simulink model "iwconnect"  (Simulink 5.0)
settings: Solver=ode45  StartTime=0  StopTime=5  MaxStep=1e-3  RelTol=1e-3
undefined symbols (not defined in the file or in its folder): fro, fso, gamo, vro, wmo
libraries: simulink x5

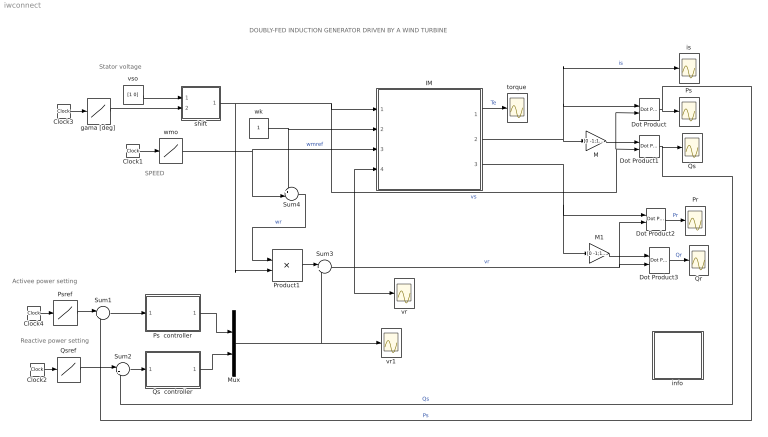
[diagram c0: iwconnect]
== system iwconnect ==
  note: DOUBLY-FED INDUCTION GENERATOR DRIVEN BY A WIND TURBINE
  note: SPEED
  note: Reactive power setting
  note: Activee power setting
  note: Stator voltage
  Clock{1..4} (4 alike) : Clock
  Dot Product{,1..3} (4 alike) : simulink/Math Operations/Dot Product
  IM : Subsystem  mask{Rs=0.01, Lsl=0.1, Rr=0.02, Lm=5, Lrl=0.1, wo=2*pi*60}
      mask prompts: Rs "Stator resistance [pu]"; Lsl "Stator leakage inductance [pu]"; Rr "Rotor resistance [pu]"; Lm "Magnetizing inductance [pu]"; Lrl "Rotor leakage inductance [pu]"; wo "base frequency [rad/s]"
  M : Gain  Gain=[0 -1;1 0]  Multiplication=Matrix(K*u)
  M1 : Gain  Gain=[0 -1;1 0]  Multiplication=Matrix(K*u)
  Mux : Mux  Inputs=2
  Pr : Scope
  Product1 : Product
  Ps : Scope
  Ps  controller : Subsystem  mask{Kp=.07, Ki=10, sat=10}
      mask prompts: Kp "Proportional gain (Kp)"; Ki "Integral gain (Ki)"; sat "Saturation limit [pu]"
      mask help: Proportional-Integral Speed Controller
  Psref : Lookup  InputValues=[0 2 2.01 30 ]  OutputValues=[0 0 -1 -1]
  Qr : Scope
  Qs : Scope
  Qs  controller : Subsystem  mask{Kp=.07, Ki=10, sat=1000}
      mask prompts: Kp "Proportional gain (Kp)"; Ki "Integral gain (Ki)"; sat "Saturation limit [pu]"
      mask help: Proportional-Integral Speed Controller
  Qsref : Lookup  InputValues=[0 3 3.01 10 ]  OutputValues=[0 0 .5 .5]
  Sum1 : Sum  Inputs=|+-
  Sum2 : Sum  Inputs=|++
  Sum3 : Sum  Inputs=|+-
  Sum4 : Sum  Inputs=+-|
  gama [deg] : Lookup  InputValues="[0  1 1.01 20]"  OutputValues=[gamo gamo 20 20]
  info : Subsystem
  is : Scope
  shift : Subsystem
  torque : Scope
  vr : Scope
  vr1 : Scope
  vso : Constant  Value=[1 0]
  wk : Constant
  wmo : Lookup  InputValues=[0 4 4.01 10 ]  OutputValues=[wmo wmo 1.3 1.3]
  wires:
  shift/1(vs) -> IM/1(vs), Dot Product/2, Dot Product1/2, Product1/2  "vs"
  wk/1 -> IM/2(wk), Sum4/1
  Dot Product/1 -> Ps/1, Sum1/2  "Ps"
  M/1 -> Dot Product1/1
  Dot Product1/1 -> Qs/1, Sum2/2  "Qs"
  IM/2(is) -> M/1, Dot Product/1, is/1  "is"
  Dot Product2/1 -> Pr/1  "Pr"
  M1/1 -> Dot Product3/1
  Dot Product3/1 -> Qr/1  "Qr"
  IM/3(ir) -> M1/1, Dot Product2/1
  Clock1/1 -> wmo/1
  wmo/1 -> IM/3(wm), Sum4/2  "wmref"
  IM/1(Te) -> torque/1  "Te"
  Qs  controller/1(Vsqer) -> Mux/2
  Sum2/1 -> Qs  controller/1(Qser)
  Sum1/1 -> Ps  controller/1(Pser)
  Ps  controller/1(Vsder) -> Mux/1
  Sum4/1 -> Product1/1  "wr"
  Product1/1 -> Sum3/1
  Sum3/1 -> IM/4(vr), Dot Product3/2, Dot Product2/2, vr/1  "vr"
  Mux/1 -> vr1/1, Sum3/2
  Clock4/1 -> Psref/1
  Psref/1 -> Sum1/1
  Clock2/1 -> Qsref/1
  Qsref/1 -> Sum2/1
  Clock3/1 -> gama [deg]/1
  vso/1 -> shift/1(vso)
  gama [deg]/1 -> shift/2(gama)

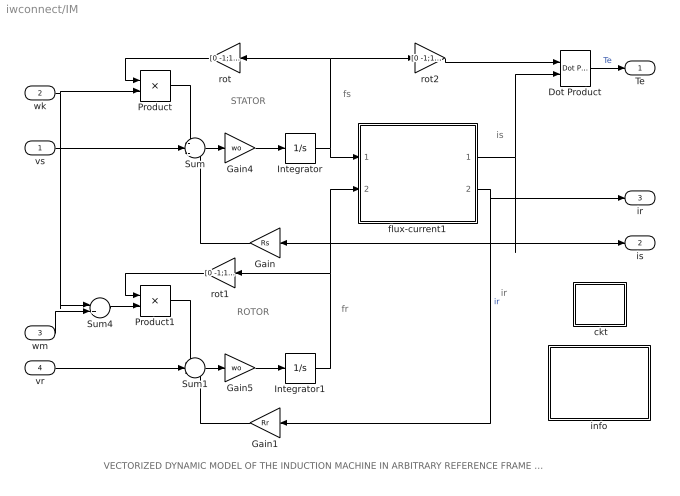
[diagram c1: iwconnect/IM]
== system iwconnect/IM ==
  note: ROTOR
  note: STATOR
  note: fs
  note: fr
  note: is
  note: VECTORIZED DYNAMIC MODEL OF THE INDUCTION MACHINE IN ARBITRARY REFERENCE FRAME (per unit formulation)
  note: ir
  vs : Inport
  wk : Inport  Port=2
  wm : Inport  Port=3
  vr : Inport  Port=4
  " ckt" : Subsystem
  Dot Product : simulink/Math Operations/Dot Product
  Gain : Gain  Orientation=left  Gain=Rs
  Gain1 : Gain  Orientation=left  Gain=Rr
  Gain4 : Gain  Gain=wo
  Gain5 : Gain  Gain=wo
  Integrator : Integrator  InitialCondition=fso
  Integrator1 : Integrator  InitialCondition=fro
  Product : Product
  Product1 : Product
  Sum : Sum  Inputs=-+-
  Sum1 : Sum  Inputs=-+-
  Sum4 : Sum  Inputs=|+-
  flux-current1 : Subsystem
  info : Subsystem
  rot : Gain  Orientation=left  Gain=[0 -1;1 0]  Multiplication=Matrix(K*u)
  rot1 : Gain  Orientation=left  Gain=[0 -1;1 0]  Multiplication=Matrix(K*u)
  rot2 : Gain  Gain=[0 -1;1 0]  Multiplication=Matrix(K*u)
  Te : Outport
  is : Outport  Port=2
  ir : Outport  Port=3
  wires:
  Gain/1 -> Sum/3
  Gain1/1 -> Sum1/3
  flux-current1/2(ir) -> Gain1/1, ir/1  "ir"
  Integrator/1 -> flux-current1/1(fs), rot/1, rot2/1
  Integrator1/1 -> flux-current1/2(fr), rot1/1
  Product1/1 -> Sum1/1
  rot1/1 -> Product1/1
  Product/1 -> Sum/1
  rot/1 -> Product/1
  rot2/1 -> Dot Product/1
  Sum4/1 -> Product1/2
  Sum/1 -> Gain4/1
  Gain4/1 -> Integrator/1
  Sum1/1 -> Gain5/1
  Gain5/1 -> Integrator1/1
  flux-current1/1(is) -> Gain/1, is/1, Dot Product/2
  Dot Product/1 -> Te/1  "Te"
  vs/1 -> Sum/2
  wk/1 -> Product/2, Sum4/1
  wm/1 -> Sum4/2
  vr/1 -> Sum1/2

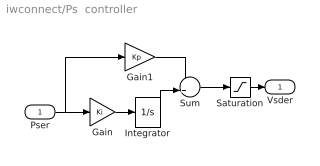
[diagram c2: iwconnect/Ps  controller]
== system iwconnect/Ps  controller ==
  Pser : Inport
  Gain : Gain  Gain=Ki
  Gain1 : Gain  Gain=Kp
  Integrator : Integrator  InitialCondition=vro(1)  LimitOutput=on  UpperSaturationLimit=sat  LowerSaturationLimit=-sat
  Saturation : Saturate  UpperLimit=sat  LowerLimit=-sat
  Sum : Sum
  Vsder : Outport  InitialOutput=0
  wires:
  Integrator/1 -> Sum/2
  Gain1/1 -> Sum/1
  Gain/1 -> Integrator/1
  Pser/1 -> Gain/1, Gain1/1
  Sum/1 -> Saturation/1
  Saturation/1 -> Vsder/1

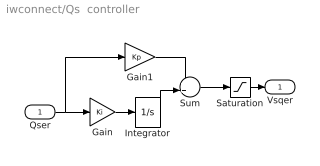
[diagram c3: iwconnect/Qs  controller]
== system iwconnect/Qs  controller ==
  Qser : Inport
  Gain : Gain  Gain=Ki
  Gain1 : Gain  Gain=Kp
  Integrator : Integrator  InitialCondition=vro(2)  LimitOutput=on  UpperSaturationLimit=sat  LowerSaturationLimit=-sat
  Saturation : Saturate  UpperLimit=sat  LowerLimit=-sat
  Sum : Sum
  Vsqer : Outport  InitialOutput=0
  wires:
  Saturation/1 -> Vsqer/1
  Sum/1 -> Saturation/1
  Qser/1 -> Gain1/1, Gain/1
  Gain/1 -> Integrator/1
  Gain1/1 -> Sum/1
  Integrator/1 -> Sum/2

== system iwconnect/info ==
  note: The induction machine is modeled in vectorized form in the synchronous frame . The d-axis is aligned with the stator space voltage vector. The injected rotor voltages (at slip frequency) are derived from PI controllers that regulate the active and reactive powers delivered by the generator. The speed is adjusted by the turbine pitch control to maximize the power generated at a given wind speed. The whole system is described by parameters expressed in per unit. The machine representations are based on the motor convention; consequently in the generator mode of operation, such quantities as Ps, Qs, Tw, Te are negative (with wm>0) while Pr is positive for subsynchronous operation and negative for oversynchronous mode. Before running this model, must be run in order to establish the initial conditions when the generator stator is disconnected from the grid.
  note: Doubly-Fed Induction Generator driven by a Wind Turbine

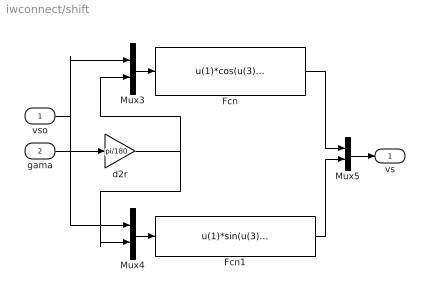
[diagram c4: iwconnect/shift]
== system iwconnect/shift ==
  vso : Inport
  gama : Inport  Port=2
  Fcn : Fcn  Expr=u(1)*cos(u(3))-u(2)*sin(u(3))
  Fcn1 : Fcn  Expr=u(1)*sin(u(3))+u(2)*cos(u(3))
  Mux3 : Mux  Inputs=2
  Mux4 : Mux  Inputs=2
  Mux5 : Mux  Inputs=2
  d2r : Gain  Gain=pi/180  Multiplication=Matrix(K*u)
  vs : Outport
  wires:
  Mux5/1 -> vs/1
  Fcn/1 -> Mux5/1
  Fcn1/1 -> Mux5/2
  gama/1 -> d2r/1
  vso/1 -> Mux4/1, Mux3/1
  Mux4/1 -> Fcn1/1
  Mux3/1 -> Fcn/1
  d2r/1 -> Mux4/2, Mux3/2

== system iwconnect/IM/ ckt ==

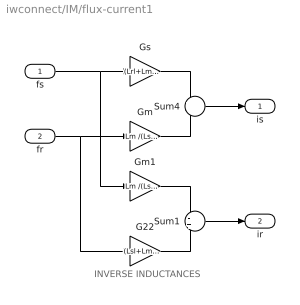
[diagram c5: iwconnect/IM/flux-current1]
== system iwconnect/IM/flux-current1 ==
  note: INVERSE INDUCTANCES
  fs : Inport
  fr : Inport  Port=2
  G22 : Gain  Gain=(Lsl+Lm )/(Lsl*Lrl+Lsl*Lm+Lrl*Lm)
  Gm : Gain  Gain=Lm /(Lsl*Lrl+Lsl*Lm+Lrl*Lm)
  Gm1 : Gain  Gain=Lm /(Lsl*Lrl+Lsl*Lm+Lrl*Lm)
  Gs : Gain  Gain=(Lrl+Lm) /(Lsl*Lrl+Lsl*Lm+Lrl*Lm)
  Sum1 : Sum  Inputs=-+
  Sum4 : Sum  Inputs=+-
  is : Outport
  ir : Outport  Port=2
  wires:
  fs/1 -> Gs/1, Gm1/1
  Gs/1 -> Sum4/1
  fr/1 -> Gm/1, G22/1
  Gm/1 -> Sum4/2
  Sum4/1 -> is/1
  Gm1/1 -> Sum1/1
  G22/1 -> Sum1/2
  Sum1/1 -> ir/1

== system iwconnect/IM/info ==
  note: Mathematical model of the induction machine. Space vector formulation in an arbitrary dq common reference frame. Per unit description.
  note: Electrical system equations: vs = Rs is + 1/wo (dfs/dt) + wk M(pi/2) fs vr = Rr ir + 1/wo (dfr/dt) + (wk - wm) M(pi/2) fr where the variables i, v, and f are 2-dimensional space vectors; for instance is = [ids iqs] and so forth, wk is the speed of the reference frame, wm the rotor speed, and M(pi/2)represents a 90o space rotator namely M(pi/2) = [0 -1;1 0] The flux linkage current relations are: fs = Ls is + Lm ir fr = Lm is + Lr ir where Ls =Lm +Lsl and Lr = Lm +Lrl Mechanical system equations: Te = 2H (dwm/dt ) + Bm wm + Tl where Te = fs (cross) is = M(pi/2) fs (dot) is = fds iqs - fqs ids = fs x is = M(pi/2) fs . is = ir x fr = Lm (ir x is) = Lm/Lr (fr x is) = 1/Lm' (fr x fs) Lm' =Lm c/(1-c) c = 1 - Lm^2/(Ls Lr)
